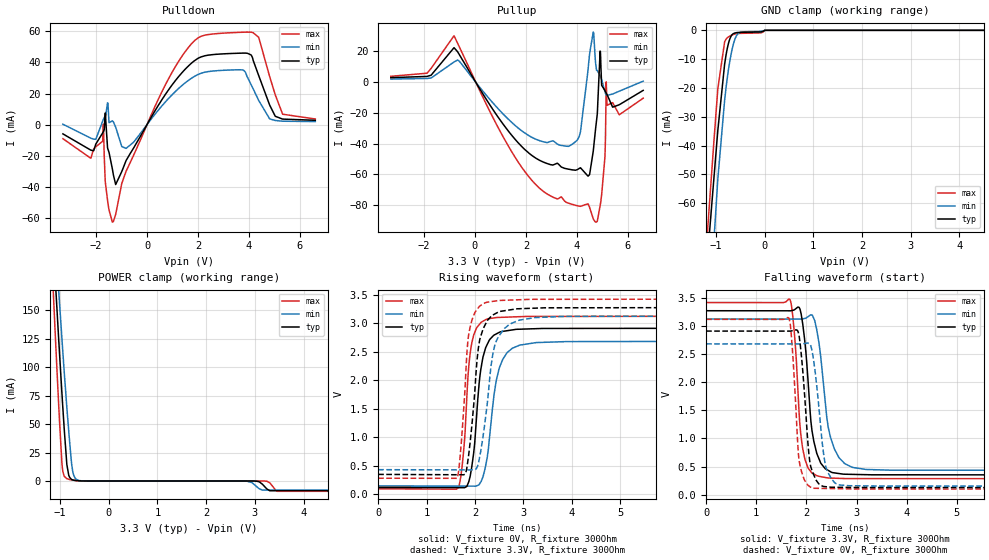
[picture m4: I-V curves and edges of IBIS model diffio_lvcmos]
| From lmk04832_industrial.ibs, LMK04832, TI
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|   diffio_lvcmos Model
[Model]   diffio_lvcmos
Model_type   I/O
Polarity   Non-Inverting
Enable   Active-High
Vinl = 0.4
Vinh = 1.2
Vmeas = 1.65
Vref = 0
Cref = 2pF
Rref = 100000
|   typ   min   max
C_comp   1.613pF   1.569pF   1.681pF
|  Where Nom  PVT is Nominal Process,   3.3V,  25C
|   Fast PVT is Strong Process,   3.45V, -40C
|   Slow PVT is Weak Process,   3.15V, 85C
[Model spec]
|subparameter
Vinl   0.400   0.370   0.430
Vinh   1.200   1.170   1.230
[Voltage Range]   3.3   3.15   3.45
|Junction Temperature
[Temperature Range]   25   85   -40
[Pullup Reference]   3.3   3.15   3.45
[Pulldown Reference]   0   0   0
[Power Clamp Reference]   3.3   3.15   3.45
[GND Clamp Reference]   0   0   0
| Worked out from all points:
|   slope of the pulldown table from 0 to 0.495 V, typ, clamps not added: 36.1 ohm
|   slope of the pullup table from 0 to 0.495 V, typ, clamps not added: 37.3 ohm
|   GND clamp passes 1 mA (typ) near -0.62 V on its own axis
|   POWER clamp passes 1 mA (typ) near -0.74 V on its own axis
|   falling waveform, V_fixture 3.3V, R_fixture 300Ohm: 20-80 % time 179ps typ, 232ps min, 144ps max; typ from 3.28 V to 0.35 V
|   rising waveform, V_fixture 0V, R_fixture 300Ohm: 20-80 % time 188ps typ, 236ps min, 149ps max; typ from 0.122 V to 2.92 V
|   rising waveform, V_fixture 3.3V, R_fixture 300Ohm: 20-80 % time 191ps typ, 243ps min, 151ps max; typ from 0.35 V to 3.28 V
|   falling waveform, V_fixture 0V, R_fixture 300Ohm: 20-80 % time 142ps typ, 178ps min, 117ps max; typ from 2.92 V to 0.122 V
[Pulldown]
|   Voltage   I(typ)   I(min)   I(max)
-3.3V     -6.006mA   194uA      -9.098mA
-2.21V    -16.42mA   -8.741mA   -21.65mA
-1.71V    -4.314mA   3.419mA    301.6uA
-1.63V    7.432mA    5.598mA    -37.88mA
-1.32V    -32.39mA   1.748mA    -62.47mA
-820mV    -23.14mA   -15.33mA   -30.01mA
960mV     25.01mA    18.8mA     32.98mA
2.82V     45.38mA    34.79mA    58.68mA
3.8V      46.02mA    34.79mA    59.49mA
4.38V     31.56mA    15.52mA    56.22mA
5.32V     3.518mA    2.159mA    6.662mA
6.6V      2.747mA    1.933mA    3.601mA
[GND Clamp]
|   Voltage   I(typ)   I(min)   I(max)
-3.3V     -880.2mA   -824.9mA   -955.5mA
-1.18V    -80.5mA    -122.1mA   -71.85mA
-1.04V    -51.39mA   -73.25mA   -38.58mA
-960mV    -34.84mA   -51.71mA   -20.4mA
-820mV    -11.74mA   -24.32mA   -3.983mA
-730mV    -3.862mA   -12.43mA   -2.166mA
-670mV    -1.608mA   -6.896mA   -1.634mA
-620mV    -991.5uA   -3.63mA    -1.335mA
-570mV    -794.2uA   -1.677mA   -1.162mA
-500mV    -706.1uA   -676.8uA   -1.062mA
0V        0A         0A         0A
6.6V      0A         0A         0A
[Pullup]
|   Voltage   I(typ)   I(min)   I(max)
-3.3V     2.772mA    1.857mA    3.653mA
-820mV    22.21mA    12.93mA    29.97mA
1.84V     -41.99mA   -31.78mA   -55.5mA
3.66V     -56.56mA   -41.78mA   -78.6mA
4.14V     -55.7mA    -32.31mA   -80.7mA
4.64V     -44.96mA   32.33mA    -88.76mA
4.75V     -27.75mA   9.99mA     -91mA
4.91V     20mA       4.176mA    -80.32mA
5.1V      -5.608mA   -6.328mA   -48.47mA
5.15V     -7.327mA   -8.5mA     18.01uA
5.66V     -14.81mA   -6.007mA   -21.32mA
6.6V      -5.48mA    491.1uA    -10.55mA
[POWER Clamp]
|   Voltage   I(typ)   I(min)   I(max)
-3.3V     1.944A     1.741A     2.257A
-1.23V    279.5mA    301.8mA    251.5mA
-1.11V    186.9mA    221.6mA    140.1mA
-1.07V    156.6mA    195.3mA    104.1mA
-1.01V    112.1mA    156.2mA    52.47mA
-960mV    76.51mA    124.5mA    14.98mA
-920mV    49.82mA    99.77mA    4.868mA
-860mV    14.5mA     64.71mA    2.062mA
-820mV    4.859mA    43.26mA    1.488mA
-740mV    963.9uA    8.663mA    758.6uA
-610mV    149uA      399.9uA    139uA
6.6V      -8.594mA   -8.021mA   -9.078mA
[Ramp]
R_load = 300
|   typ   min   max
dV/dt_r   1.67579/1.86928e-10   1.52294/2.35793e-10   1.81631/1.48689e-10
dV/dt_f   1.75689/1.78561e-10   1.61863/2.29298e-10   1.88497/1.43253e-10
[Falling Waveform]
V_fixture = 3.3V
V_fixture_min = 3.15V
V_fixture_max = 3.45V
R_fixture = 300Ohm
C_fixture = 0F
|   Time   V(typ)   V(min)   V(max)
0s        3.278V     3.13V      3.424V
1.671ns   3.277V     3.129V     3.478V
1.762ns   3.295V     3.129V     2.862V
1.865ns   3.319V     3.129V     1.306V
1.917ns   3.101V     3.131V     876.2mV
2.092ns   1.29V      3.204V     405.6mV
2.208ns   732.6mV    2.93V      337.7mV
2.471ns   413.3mV    1.058V     294.9mV
2.917ns   360.4mV    486.1mV    285.2mV
10ns      349.6mV    432.4mV    282.7mV
[Rising Waveform]
V_fixture = 0V
V_fixture_min = 0V
V_fixture_max = 0V
R_fixture = 300Ohm
C_fixture = 0F
|   Time   V(typ)   V(min)   V(max)
0s        122mV      148.4mV    96.76mV
1.651ns   116.8mV    144.5mV    113.2mV
1.758ns   116.5mV    144.3mV    701.2mV
1.859ns   196.8mV    144.1mV    2.124V
1.922ns   428.9mV    143.9mV    2.605V
2.101ns   2.078V     193.7mV    2.992V
2.227ns   2.586V     540.2mV    3.067V
2.492ns   2.837V     2.189V     3.102V
2.917ns   2.896V     2.615V     3.115V
10ns      2.915V     2.687V     3.124V
[Rising Waveform]
V_fixture = 3.3V
V_fixture_min = 3.15V
V_fixture_max = 3.45V
R_fixture = 300Ohm
C_fixture = 0F
|   Time   V(typ)   V(min)   V(max)
0s        349.6mV    432.5mV    282.7mV
1.627ns   343.5mV    429.3mV    281mV
1.709ns   343.2mV    429.2mV    833.2mV
1.816ns   402.5mV    429mV      2.25V
1.87ns    701.2mV    428.8mV    2.811V
2.069ns   2.567V     549.2mV    3.273V
2.208ns   2.973V     1.284V     3.359V
2.409ns   3.164V     2.617V     3.39V
2.917ns   3.255V     3.055V     3.412V
10ns      3.278V     3.13V      3.424V
[Falling Waveform]
|Gnd
V_fixture = 0V
V_fixture_min = 0V
V_fixture_max = 0V
R_fixture = 300Ohm
C_fixture = 0F
|   Time   V(typ)   V(min)   V(max)
0s        2.915V     2.687V     3.124V
1.649ns   2.914V     2.686V     3.148V
1.718ns   2.921V     2.686V     2.622V
1.853ns   2.831V     2.686V     619.7mV
1.928ns   2.202V     2.691V     343.2mV
2.052ns   703.5mV    2.692V     153.3mV
2.108ns   441mV      2.586V     117.3mV
2.377ns   141.5mV    533.6mV    109.1mV
2.637ns   129.9mV    176.2mV    104.9mV
10ns      122mV      148.4mV    96.76mV
